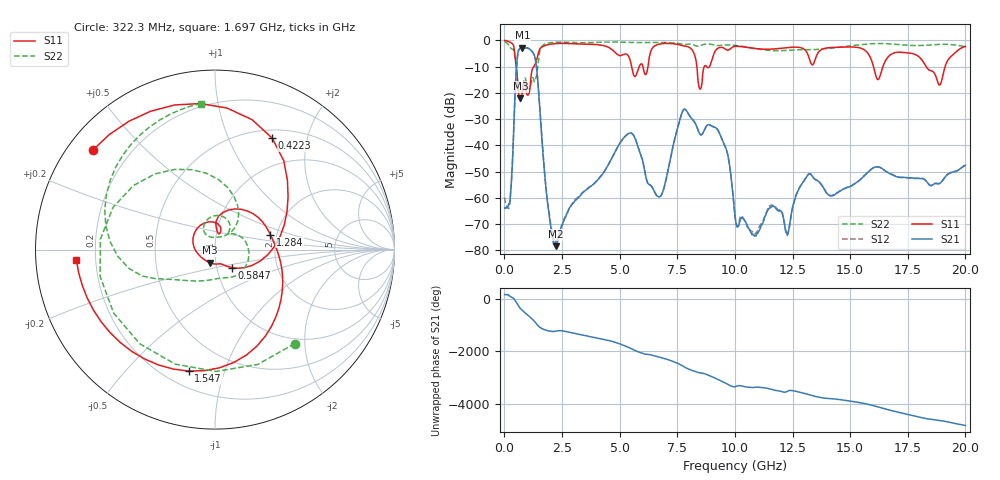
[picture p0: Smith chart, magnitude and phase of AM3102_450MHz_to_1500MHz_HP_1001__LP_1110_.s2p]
!Agilent Technologies,E8364B,MY43040894,A.07.50.67
!Agilent E8364B: A.07.50.67
!Date: Thursday, January 11, 2018 06:05:53
!Correction: S11(Full 2 Port(1,2))
!S21(Full 2 Port(1,2))
!S12(Full 2 Port(1,2))
!S22(Full 2 Port(1,2))
!S2P File: Measurements: S11, S21, S12, S22:
# Hz S  dB  R 50
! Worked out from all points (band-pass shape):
!   1601 points, 10 MHz to 20 GHz, reference 50 ohm
!   highest |S21| = -2.76 dB at 784.6 MHz (marker M1); lowest = -78.4 dB at 2.221 GHz (marker M2)
!   |S21| within 3 dB of the highest: 573.1 MHz to 1.3 GHz (727.4 MHz wide, 77.6 % of centre)
!   lowest |S11| = -22.1 dB at 697.2 MHz (marker M3), VSWR 1.17, Z = 46.7 - j6.87 ohm
!   |S11| at or under -10 dB: 515 MHz to 1.276 GHz (761 MHz wide, 85 % of centre); 16.01 GHz to 16.42 GHz (410.8 MHz wide, 2.53 % of centre); 18.3 GHz to 19.12 GHz (825 MHz wide, 4.41 % of centre)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
!   |S22| runs from -23.3 to -0.5 dB; largest |S21 - S12| = 0.0017
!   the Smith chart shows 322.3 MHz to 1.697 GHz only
!   S11 on the Smith chart (normalised r, x): 322.3 MHz: 0.07, +0.35; 422.3 MHz: 0.60, +1.46; 584.7 MHz: 1.18, -0.24; 1.284 GHz: 1.85, +0.35; 1.547 GHz: 0.29, -0.76; 1.697 GHz: 0.13, -0.04
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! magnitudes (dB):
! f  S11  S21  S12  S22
! 10 MHz  -0.1  -63.8  -59.9  -0.5
! 322.3 MHz  -1.1  -51.2  -51.1  -3.3
! 422.3 MHz  -3.1  -29.3  -29.6  -4.2
! 584.7 MHz  -17.2  -5.0  -5.0  -17.3
! 697.2 MHz  -22.1  -2.9  -2.9  -23.3
! 784.6 MHz  -19.4  -2.8  -2.8  -19.7
! 1.284 GHz  -9.9  -5.4  -5.4  -15.6
! 1.547 GHz  -3.2  -27.4  -27.4  -3.7
! 1.697 GHz  -2.2  -45.7  -45.7  -1.7
! 2.221 GHz  -1.3  -78.4  -76.6  -0.7
! 3.346 GHz  -1.4  -58.6  -58.4  -0.9
! 5.457 GHz  -7.7  -35.3  -35.3  -0.8
! 6.682 GHz  -1.5  -59.6  -59.6  -0.8
! 7.844 GHz  -2.2  -26.3  -26.3  -1.6
! 8.493 GHz  -18.6  -35.8  -35.9  -2.1
! 9.33 GHz  -2.8  -35.4  -35.4  -2.0
! 10.01 GHz  -2.3  -66.8  -67.0  -1.9
! 12.28 GHz  -2.8  -73.9  -74.1  -3.8
! 13.34 GHz  -9.3  -51.5  -51.6  -3.6
! 16.68 GHz  -6.1  -50.6  -50.5  -1.3
! 18.88 GHz  -17.0  -54.4  -54.6  -1.5
! 20 GHz  -2.4  -47.6  -47.6  -2.3
